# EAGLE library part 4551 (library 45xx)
Quad 2-channel analog MULTIPLEXER/DEMULTIPLEXER
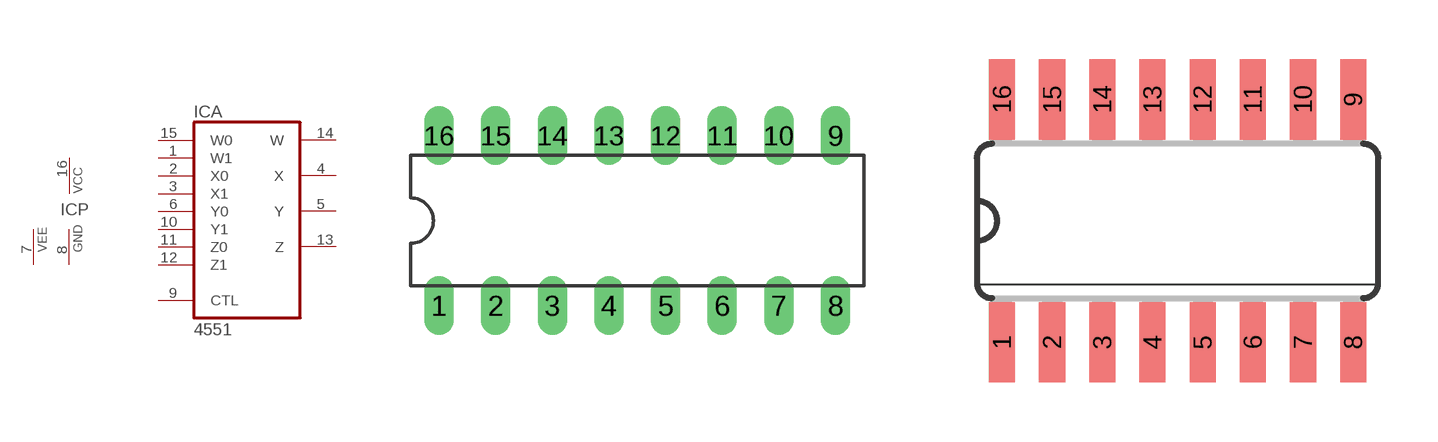
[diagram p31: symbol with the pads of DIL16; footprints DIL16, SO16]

Designator prefix IC; gates A=4551 P=PWR+VEE

## 4551N  [DIL16]
1  A:W1
2  A:X0
3  A:X1
4  A:X
5  A:Y
6  A:Y0
7  P:VEE  pwr
8  P:GND  pwr
9  A:CTL  in
10  A:Y1
11  A:Z0
12  A:Z1
13  A:Z
14  A:W
15  A:W0
16  P:VCC  pwr

## 4551D  [SO16]
Pads as for DIL16

## Footprint DIL16 (pad centres in mm)
Dual In Line Package
drill 0.813 long: 1 -8.89,-3.81; 2 -6.35,-3.81; 3 -3.81,-3.81; 4 -1.27,-3.81; 5 1.27,-3.81; 6 3.81,-3.81; 7 6.35,-3.81; 8 8.89,-3.81; 9 8.89,3.81; 10 6.35,3.81; 11 3.81,3.81; 12 1.27,3.81; 13 -1.27,3.81; 14 -3.81,3.81; 15 -6.35,3.81; 16 -8.89,3.81

## Footprint SO16 (pad centres in mm)
Small Outline package 150 mil
smd 0.66 x 2.032: 1 -4.445,-3.073; 2 -3.175,-3.073; 3 -1.905,-3.073; 4 -0.635,-3.073; 5 0.635,-3.073; 6 1.905,-3.073; 7 3.175,-3.073; 8 4.445,-3.073; 9 4.445,3.073; 10 3.175,3.073; 11 1.905,3.073; 12 0.635,3.073; 13 -0.635,3.073; 14 -1.905,3.073; 15 -3.175,3.073; 16 -4.445,3.073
